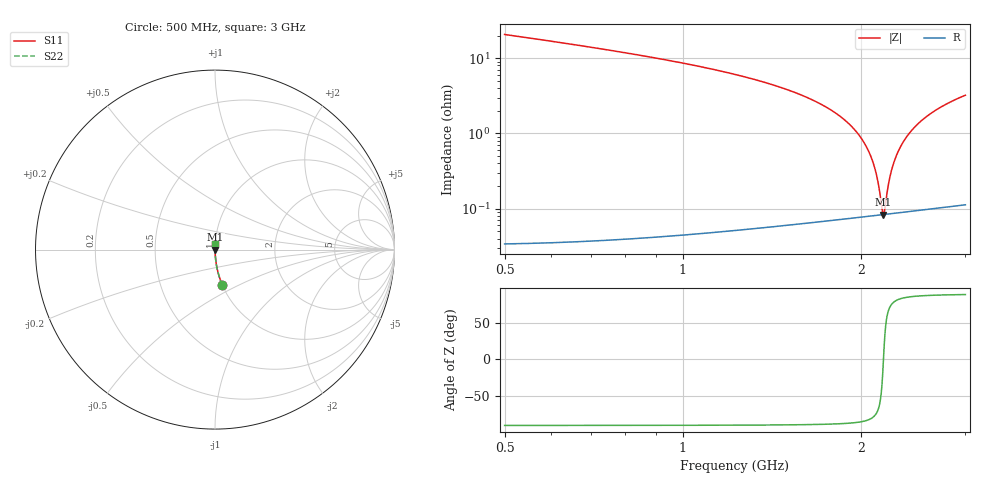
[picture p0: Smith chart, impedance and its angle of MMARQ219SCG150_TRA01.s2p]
! MMARQ219SCG150_TRA01  S-PARAMETER MODEL  ( General Type )
! Model Generated by TAIYO YUDEN Corporation (http://www.ty-top.com)
! Version 1.0
! TAIYO YUDEN Control No. 150609
! Copyright(c) 2015 TAIYO YUDEN CO.,LTD. All Rights Reserved.
! Product Description (link to TY-COMPAS)
! https://ds.yuden.co.jp/TYCOMPAS/or/detail?pn=MMARQ219SCG150JTRA01&u=M
! Products Name : Multilayer Ceramic Capacitors
! Characteristics :
!  Capacitance : 15 pF , Rated Voltage : 250V , TCC : CG / C0G
!  Case Size : 2.0 x 1.25 / 0.079 x 0.049 [mm/inch] , Thickness : 0.85 / 0.033 [mm/inch]
!  (Conditions: Temperature = 25 degC , DC Bias Current/Voltage = 0A / 0V)
! External Node Assignments :
!  1  o---| |---o  2
! GND o---------o GND
! Frequency Range : 500MHz  -  3GHz  [ 401 STEP ]
# MHz S RI R 50
! Freq[MHz].  S11 Real  S11 Imag  S21 Real  S21 Imag  S12 Real  S12 Imag  S22 Real  S22 Imag
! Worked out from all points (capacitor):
!   401 points, 500 MHz to 3 GHz, reference 50 ohm
!   read as one part in series: C = 14.6 pF near 512.5 MHz
!   lowest |Z| = 83.6 mohm at 2.181 GHz (marker M1)
!   series resonance near 2.182 GHz, so ESL is about 360 pH
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500  0.0412 -0.198  0.9588 0.198  0.9588 0.198  0.0412 -0.198
918.75  0.00984 -0.0965  0.9902 0.0965  0.9902 0.0965  0.00984 -0.0965
1337.5  0.00312 -0.0506  0.9969 0.0506  0.9969 0.0506  0.00312 -0.0506
1568.75  0.00174 -0.0334  0.9983 0.0334  0.9983 0.0334  0.00174 -0.0334
1750  0.00118 -0.0221  0.9988 0.0221  0.9988 0.0221  0.00118 -0.0221
1925  0.000902 -0.0125  0.9991 0.0125  0.9991 0.0125  0.000902 -0.0125
1987.5  0.000854 -0.00928  0.9991 0.00928  0.9991 0.00928  0.000854 -0.00928
2043.75  0.000829 -0.00649  0.9992 0.00649  0.9992 0.00649  0.000829 -0.00649
2087.5  0.000822 -0.00438  0.9992 0.00438  0.9992 0.00438  0.000822 -0.00438
2118.75  0.000822 -0.0029  0.9992 0.0029  0.9992 0.0029  0.000822 -0.0029
2143.75  0.000825 -0.00174  0.9992 0.00174  0.9992 0.00174  0.000825 -0.00174
2168.75  0.000831 -0.000585  0.9992 0.000585  0.9992 0.000585  0.000831 -0.000585
2181.25  0.000835 -1.32e-05  0.9992 1.32e-05  0.9992 1.32e-05  0.000835 -1.32e-05
2193.75  0.00084 0.000555  0.9992 -0.000555  0.9992 -0.000555  0.00084 0.000555
2225  0.000854 0.00196  0.9991 -0.00196  0.9991 -0.00196  0.000854 0.00196
2250  0.000869 0.00307  0.9991 -0.00307  0.9991 -0.00307  0.000869 0.00307
2281.25  0.00089 0.00444  0.9991 -0.00444  0.9991 -0.00444  0.00089 0.00444
2312.5  0.000915 0.0058  0.9991 -0.0058  0.9991 -0.0058  0.000915 0.0058
2425  0.00103 0.0105  0.999 -0.0105  0.999 -0.0105  0.00103 0.0105
2587.5  0.00127 0.017  0.9987 -0.017  0.9987 -0.017  0.00127 0.017
2775  0.00163 0.0241  0.9984 -0.0241  0.9984 -0.0241  0.00163 0.0241
3000  0.00216 0.0321  0.9978 -0.0321  0.9978 -0.0321  0.00216 0.0321
